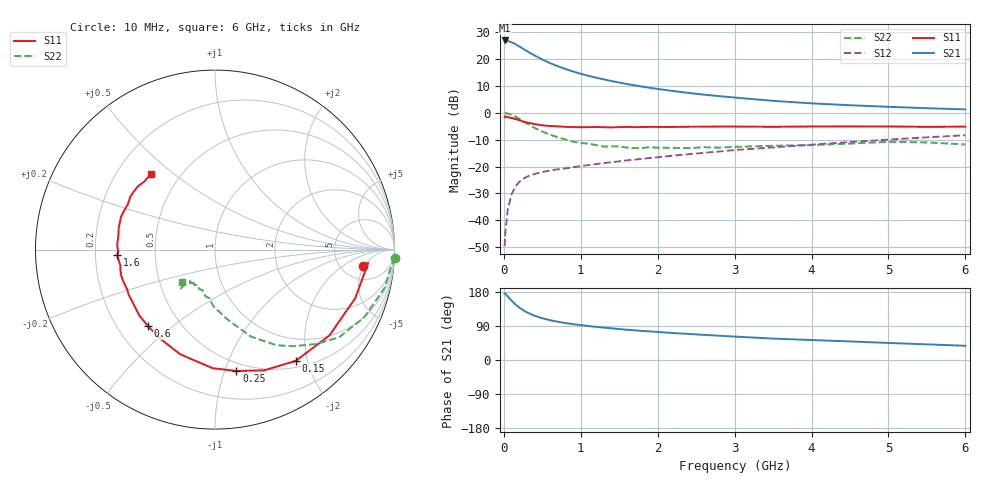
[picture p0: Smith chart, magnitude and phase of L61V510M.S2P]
!  INFINEON TECHNOLOGIES Small Signal Semiconductors
! BFR380L3 , Si-NPN RF-Transistor in TSLP-3-1
!  Vce=1.5 V,  Ic=10 mA
! Common Emitter S-Parameters:  07. March 2005
#  GHz  S  MA  R  50
! f  S11  S21  S12  S22
! GHz  Mag  Ang  Mag  Ang  Mag  Ang  Mag  Ang
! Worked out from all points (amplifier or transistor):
!   36 points, 10 MHz to 6 GHz, reference 50 ohm
!   highest |S21| = 26.9 dB at 10 MHz (marker M1)
!   |S21| within 3 dB of that: start of sweep to 246.1 MHz
!   unconditionally stable (mu >= 1): 2.183 GHz to 4.842 GHz
!   at 250 MHz: K = 0.26, MSG = 24.2 dB, |S12| = -24.6 dB
!   at 1.4 GHz: K = 0.88, MSG = 15.1 dB, |S12| = -18.4 dB
!   at 6 GHz: K = 0.97, MSG = 4.8 dB, |S12| = -8.4 dB
!   S11 on the Smith chart (normalised r, x): 10 MHz: 7.93, -4.56; 150 MHz: 0.60, -1.81; 250 MHz: 0.43, -1.10; 600 MHz: 0.33, -0.41; 1.6 GHz: 0.29, -0.03; 6 GHz: 0.34, +0.42
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0.01  0.8273 -6.3  22.11 175.8  0.0033 83.8  1.005 -2.6
0.02  0.8566 -5.0  22 175.4  0.0059 91.1  0.9858 -5.3
0.05  0.827 -19.1  21.65 167.9  0.0156 80.9  0.9695 -12.6
0.1  0.7972 -36.9  20.43 156.9  0.0304 72.1  0.9136 -24.3
0.15  0.7659 -54.0  18.9 146.8  0.0422 64.9  0.8469 -35.2
0.2  0.7266 -67.8  17.15 138.4  0.0518 60.2  0.7702 -43.1
0.25  0.6868 -80.0  15.53 131.7  0.0589 54.8  0.6916 -51.1
0.3  0.661 -91.1  14 125.7  0.0648 51.7  0.6333 -57.3
0.4  0.6147 -108.3  11.6 116.7  0.0727 47.6  0.5225 -67.7
0.5  0.5833 -121.0  9.788 110.3  0.079 46.2  0.4459 -74.0
0.6  0.5665 -131.4  8.373 105.0  0.0842 45.2  0.3928 -80.2
0.8  0.5461 -146.1  6.517 97.5  0.0923 45.7  0.3186 -91.1
0.9  0.5427 -152.3  5.837 94.6  0.0969 46.6  0.2891 -94.9
1.1  0.5403 -160.5  4.863 89.6  0.1064 48.2  0.2664 -101.0
1.4  0.5348 -170.5  3.879 83.7  0.1196 50.7  0.2378 -108.3
1.6  0.5451 -176.7  3.421 79.9  0.1301 52.1  0.2247 -116.1
2.2  0.5442 171.5  2.537 71.2  0.1594 55.4  0.2226 -121.4
2.8  0.5541 161.5  2.036 64.0  0.1903 57.7  0.2245 -128.7
3.5  0.5474 152.2  1.664 56.5  0.2267 58.0  0.2433 -129.8
4.5  0.5565 144.9  1.379 49.0  0.2855 58.6  0.2669 -131.0
5.5  0.5468 136.0  1.215 41.3  0.3487 56.4  0.2806 -132.4
6  0.5515 130.5  1.154 37.5  0.3821 54.8  0.2573 -135.0
